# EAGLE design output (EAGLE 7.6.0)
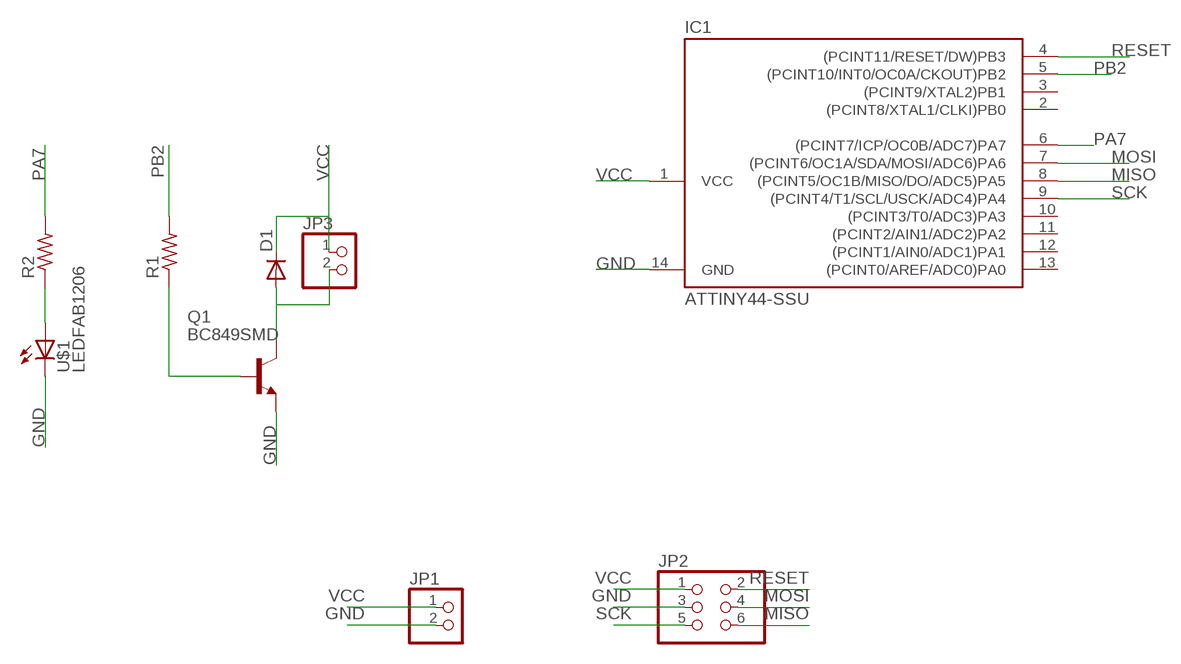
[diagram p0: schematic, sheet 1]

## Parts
D1  DIODESOD123  [SOD123]
IC1  ATTINY44-SSU  [SOIC14]
JP1  PINHD-1X2  [1X02]
JP2  PINHD-2X3  [2X03]
JP3  PINHD-1X2  [1X02]
Q1  BC849SMD  [SOT23-BEC]
R1  RES-US1206FAB  [R1206FAB]
R2  RES-US1206FAB  [R1206FAB]
U$1  LEDFAB1206  [LED1206FAB]

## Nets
GND: IC1.14(GND) JP1.2 JP2.3 Q1.E U$1.2(C)
MISO: IC1.8((PCINT5/OC1B/MISO/DO/ADC5)PA5) JP2.6
MOSI: IC1.7((PCINT6/OC1A/SDA/MOSI/ADC6)PA6) JP2.4
N$1: R2.1 U$1.1(A)
N$2: Q1.B R1.1
N$3: D1.ANODE(A) JP3.2 Q1.C
PA7: IC1.6((PCINT7/ICP/OC0B/ADC7)PA7) R2.2
PB2: IC1.5((PCINT10/INT0/OC0A/CKOUT)PB2) R1.2
RESET: IC1.4((PCINT11/RESET/DW)PB3) JP2.2
SCK: IC1.9((PCINT4/T1/SCL/USCK/ADC4)PA4) JP2.5
VCC: D1.CATHODE(C) IC1.1(VCC) JP1.1 JP2.1 JP3.1
Unconnected: IC1.2((PCINT8/XTAL1/CLKI)PB0) IC1.3((PCINT9/XTAL2)PB1) IC1.10((PCINT3/T0/ADC3)PA3) IC1.11((PCINT2/AIN1/ADC2)PA2) IC1.12((PCINT1/AIN0/ADC1)PA1) IC1.13((PCINT0/AREF/ADC0)PA0)

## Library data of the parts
D1 = fab:DIODE: DIODE
IC1 = fab:ATTINY44
JP1 JP3 = pinhead:PINHD-1X2: PIN HEADER
JP2 = pinhead:PINHD-2X3: PIN HEADER
Q1 = transistor-npn:BC849*: NPN Transistor
R1 R2 = fab:RES-US: Resistor (US Symbol)
U$1 = fab:LED: LED

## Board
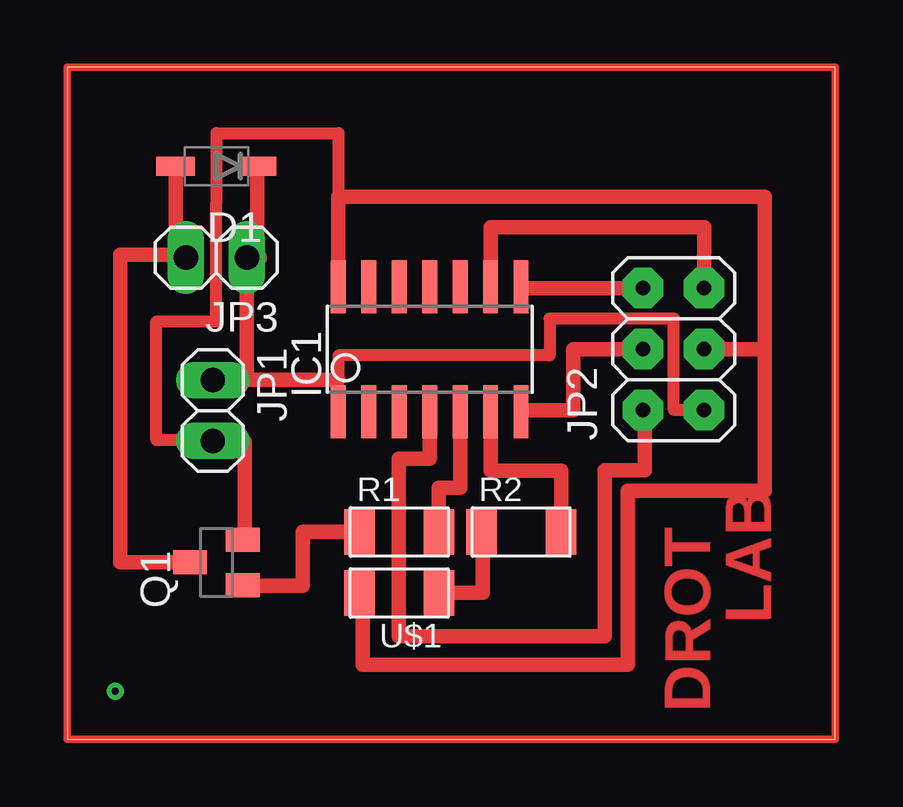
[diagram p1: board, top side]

Size 32 x 28 mm. Coordinates in mm from the lower left corner, seen from the top.
Outline: 0,0 32,0 32,28 0,28 0,0
Copper layers (1*16): Top 0.035mm / dielectric 1.5mm / Bottom 0.035mm
Design rules "default": minimum track width 10mil, minimum drill 24mil, track to track 8mil, track to pad 8mil, pad to pad 8mil, via to via 8mil, smd to smd 8mil, copper to edge 40mil, drill to drill 8mil, minimum pad ring 10mil, minimum via ring 8mil, stop-mask expansion 4mil, vias tented up to drill 0mil, thermal gap 10mil

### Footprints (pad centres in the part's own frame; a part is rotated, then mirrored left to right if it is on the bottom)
SOD123 = smd 1.6 x 0.8: ANODE 1.7,0; CATHODE -1.7,0
SOIC14 = smd 0.61 x 2.21: 1 -3.81,-2.603; 2 -2.54,-2.603; 3 -1.27,-2.603; 4 0,-2.603; 5 1.27,-2.603; 6 2.54,-2.603; 7 3.81,-2.603; 8 3.81,2.603; 9 2.54,2.603; 10 1.27,2.603; 11 0,2.603; 12 -1.27,2.603; 13 -2.54,2.603; 14 -3.81,2.603
1X02 = drill 1.016 long: 1 -1.27,0; 2 1.27,0
2X03 = drill 0.6 pad 1.676 octagon: 1 -2.54,-1.27; 2 -2.54,1.27; 3 0,-1.27; 4 0,1.27; 5 2.54,-1.27; 6 2.54,1.27
SOT23-BEC = smd 1 x 1.4: B -0.95,-1.1; C 0,1.1; E 0.95,-1.1
R1206FAB = smd 1.27 x 1.905: 1 -1.651,0; 2 1.651,0
LED1206FAB = smd 1.27 x 1.905: 1 -1.651,0; 2 1.651,0

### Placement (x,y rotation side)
D1  6.21,23.88 180 top
IC1  15.1,16.26 0 top
JP1  6.06,13.7 270 top
JP2  25.26,16.26 90 top
JP3  6.21,20.07 180 top
Q1  6.21,7.37 90 top
R1  13.83,8.64 0 top
R2  18.91,8.64 0 top
U$1  13.83,6.1 180 top

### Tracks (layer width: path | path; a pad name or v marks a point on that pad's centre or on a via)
GND
  Top 0.5: 7.4,8.32 7.41,8.32 7.41,12.47 3.71,12.47 3.71,17.41 6.21,17.41 6.21,22.38 6.22,22.38 6.22,25.26 11.29,25.26 11.29,22.61
  Top 0.61: JP2.3 29.06,16.26 | IC1.14 11.29,22.61 29.07,22.61 29.07,16.26 29.06,16.26 | 7.4,8.32 7.4,12.4 4.94,12.4 | U$1.2 12.3,6.1 12.3,3.1 23.36,3.1 | 23.36,3.1 23.35,3.13 | 29.06,16.26 29.06,10.35 23.36,10.35 23.36,3.1
  Top 0.813: Q1.E 7.4,8.32 | 4.94,12.4 JP1.2
MISO
  Top 0.61: JP2.6 18.91,18.8 IC1.8
MOSI
  Top 0.61: JP2.4 21.08,16.26 21.08,13.72 18.91,13.72 IC1.7
N$1
  Top 0.61: 17.3,8.64 17.3,6.1 U$1.1
  Top 0.813: R2.1 17.3,8.64
N$2
  Top 0.61: R1.1 9.8,8.64 9.8,6.4 7.31,6.4
  Top 0.813: 7.31,6.4 Q1.B
N$3
  Top 0.61: 4.51,20.07 D1.ANODE | Q1.C 2.2,7.37 2.2,20.2 4.94,20.2
  Top 0.813: 4.51,20.07 JP3.2 4.94,20.2
N$4
  Top 0.305: 0,28 32,28 32,0 0,0 0,28
N$5  (via drill 0.3 pad 0.41)
  other vias: 2,2
PA7
  Top 0.61: IC1.6 17.64,11.18 20.58,11.18 20.58,8.64
  Top 0.813: 20.58,8.64 R2.2
PB2
  Top 0.61: IC1.5 16.37,10.48 15.48,10.48 R1.2
RESET
  Top 0.61: IC1.4 15.1,11.7 13.8,11.7 13.8,4.3 22.4,4.3 22.4,11.22 24.05,11.22 24.05,13.72 JP2.2
SCK
  Top 0.61: JP2.5 26.53,21.34 17.64,21.34 IC1.9
VCC
  Top 0.5: IC1.1 11.29,14.99 11.29,16 20.1,16 20.1,17.53 25.27,17.53 25.27,13.72 JP2.1
  Top 0.61: 7.91,20.07 D1.CATHODE | JP3.1 7.48,14.99 | 7.48,14.99 JP1.1 | 11.29,14.99 7.48,14.99
  Top 0.813: JP3.1 7.91,20.07

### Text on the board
Top: LAB | DROT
